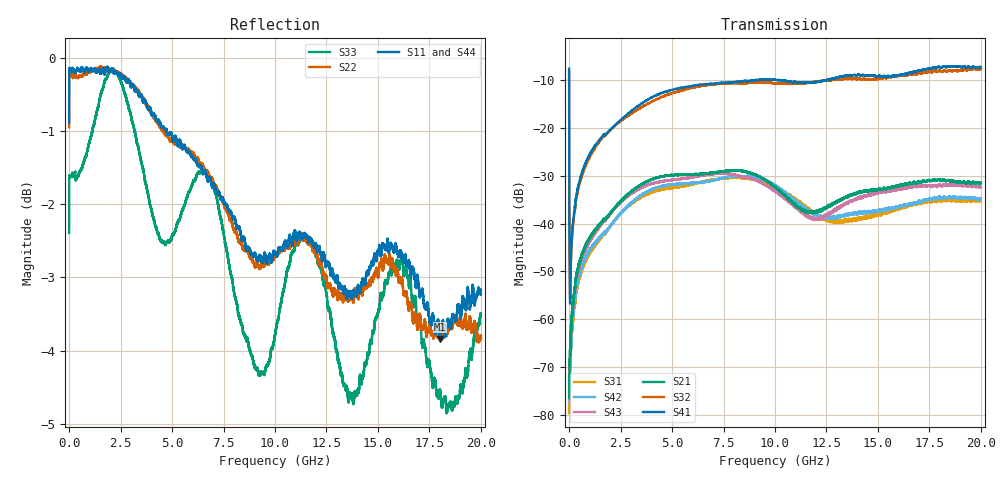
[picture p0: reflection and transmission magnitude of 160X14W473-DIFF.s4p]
!{160X14W473}
!Johanson Technology Inc.
!www.johansontechnology.com
!Test Board Conditions:
!Substrate Type  RO4350B
!Substrate Thickness  10 mil
!Substrate Dk  3.66
!TL Type: GCPW
!TL Trace Width  20 mil
!TL Gap  15 mil
!PART MODE DIFFERENTIAL
!DUT TOPOLOGY	DIFFERENTIAL 4-PORT
!Mounting Pad LxW  20x35 mil
# MHz S  dB  R 50
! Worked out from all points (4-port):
!   20001 points, 300 kHz to 20 GHz, reference 50 ohm
!   strongest paths, dB at 300 kHz, 5 GHz, 10 GHz, 15 GHz, 20 GHz:
!     S41: -7.6, -12.1, -9.9, -9.2, -7.3
!     S32: -8.3, -12.8, -10.7, -9.8, -7.6
!     S21: -72.0, -29.9, -32.3, -33.0, -31.6
!     S43: -76.2, -30.9, -33.3, -33.8, -32.3
!     S42: -77.3, -31.9, -32.0, -37.4, -34.9
!     S31: -72.8, -32.6, -32.4, -38.2, -35.3
!   lowest |S11| = -3.8 dB at 18.02 GHz (marker M1), VSWR 4.60, Z = 26.3 + j56.1 ohm
!   |S11| at or under -10 dB: nowhere
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0.3  -0.89 -155.4  -80.20 -68.0  -74.46 -29.7  -7.65 -65.1
     -71.98 2.0  -0.95 -155.6  -8.28 -65.1  -69.18 -1.7
     -72.78 -53.0  -8.26 -65.6  -2.39 -153.7  -85.93 -18.8
     -7.63 -64.9  -77.27 25.4  -76.19 1.2  -0.80 -155.6
111.298  -0.19 178.8  -60.14 70.9  -63.68 69.6  -44.63 67.9
         -60.92 65.6  -0.23 178.9  -45.41 66.3  -63.37 66.6
         -63.65 62.7  -45.38 66.5  -1.62 178.6  -61.47 74.4
         -44.62 68.1  -61.94 70.2  -61.68 73.1  -0.02 178.9
676.29  -0.15 173.9  -45.74 73.1  -48.96 70.3  -28.71 75.2
        -45.72 73.3  -0.24 172.1  -29.45 74.8  -48.36 69.4
        -49.12 70.8  -29.40 74.8  -1.46 170.6  -46.57 74.6
        -28.72 75.1  -48.13 69.4  -46.68 74.5  -0.09 171.9
3559.247  -0.57 157.2  -31.70 53.6  -34.34 43.9  -14.77 57.1
          -31.70 53.4  -0.53 158.1  -15.60 55.7  -33.95 46.5
          -34.31 44.3  -15.58 55.8  -1.49 158.4  -32.42 50.8
          -14.80 57.2  -33.94 46.5  -32.41 50.3  -0.47 156.5
12024.12  -2.58 116.0  -37.55 -8.4  -38.14 -76.8  -10.44 -9.2
          -37.59 -9.2  -2.68 118.1  -10.32 -12.5  -38.33 -71.2
          -38.13 -76.9  -10.34 -12.2  -2.70 114.2  -39.11 -16.5
          -10.41 -9.2  -38.24 -71.0  -38.95 -16.3  -2.40 114.0
18015.03  -3.84 76.6  -30.90 -27.3  -35.23 -76.1  -7.22 -35.5
          -30.88 -27.1  -3.65 81.4  -8.09 -37.4  -34.56 -73.2
          -35.12 -73.5  -8.04 -37.1  -4.55 80.5  -31.92 -25.8
          -7.32 -35.1  -34.46 -72.9  -31.94 -26.1  -3.40 81.3
20000  -3.21 67.2  -31.50 -38.6  -35.14 -87.1  -7.32 -45.8
       -31.55 -38.3  -3.84 70.9  -7.64 -46.2  -34.95 -87.3
       -35.28 -85.9  -7.62 -45.4  -3.51 62.0  -32.16 -41.1
       -7.33 -45.3  -34.87 -87.8  -32.34 -41.8  -3.31 62.8
